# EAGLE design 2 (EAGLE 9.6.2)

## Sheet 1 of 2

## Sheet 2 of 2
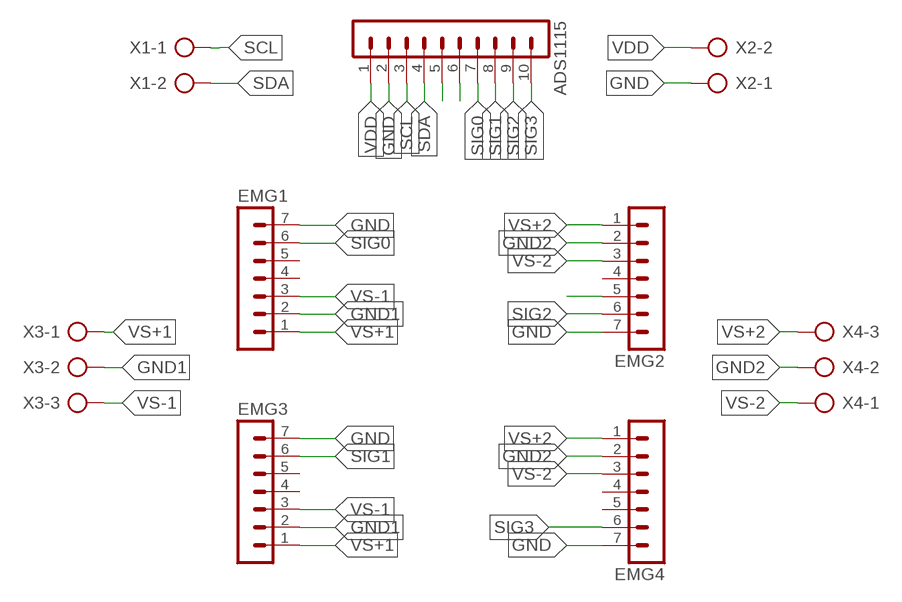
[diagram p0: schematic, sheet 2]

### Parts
ADS1115  MA10-1  [MA10-1]
EMG1  MA07-1  [MA07-1]
EMG2  MA07-1  [MA07-1]
EMG3  MA07-1  [MA07-1]
EMG4  MA07-1  [MA07-1]
X1  AK300/2  [AK300/2]
X2  AK300/2  [AK300/2]
X3  AK300/3  [AK300/3]
X4  AK300/3  [AK300/3]

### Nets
GND: ADS1115.2 EMG1.7 EMG2.7 EMG3.7 EMG4.7 X2.1
GND1: EMG1.2 EMG3.2 X3.2
GND2: EMG2.2 EMG4.2 X4.2
N$7: ADS1115.5
N$8: ADS1115.6
N$14: EMG2.5
SCL: ADS1115.3 X1.1
SDA: ADS1115.4 X1.2
SIG0: ADS1115.7 EMG1.6
SIG1: ADS1115.8 EMG3.6
SIG2: ADS1115.9 EMG2.6
SIG3: ADS1115.10 EMG4.6
VDD: ADS1115.1 X2.2
VS+1: EMG1.1 EMG3.1 X3.1
VS+2: EMG2.1 EMG4.1 X4.3
VS-1: EMG1.3 EMG3.3 X3.3
VS-2: EMG2.3 EMG4.3 X4.1
Unconnected: EMG1.4 EMG1.5 EMG2.4 EMG3.4 EMG3.5 EMG4.4 EMG4.5

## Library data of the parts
ADS1115 = con-lstb:MA10-1: PIN HEADER; OC_FARNELL: unknown; OC_NEWARK: unknown
EMG1-EMG4 = con-lstb:MA07-1: PIN HEADER; OC_FARNELL: unknown; OC_NEWARK: unknown
X1 X2 = con-ptr500:AK300/2: CONNECTOR; OC_FARNELL: unknown; OC_NEWARK: unknown
X3 X4 = con-ptr500:AK300/3: CONNECTOR; OC_FARNELL: unknown; OC_NEWARK: unknown

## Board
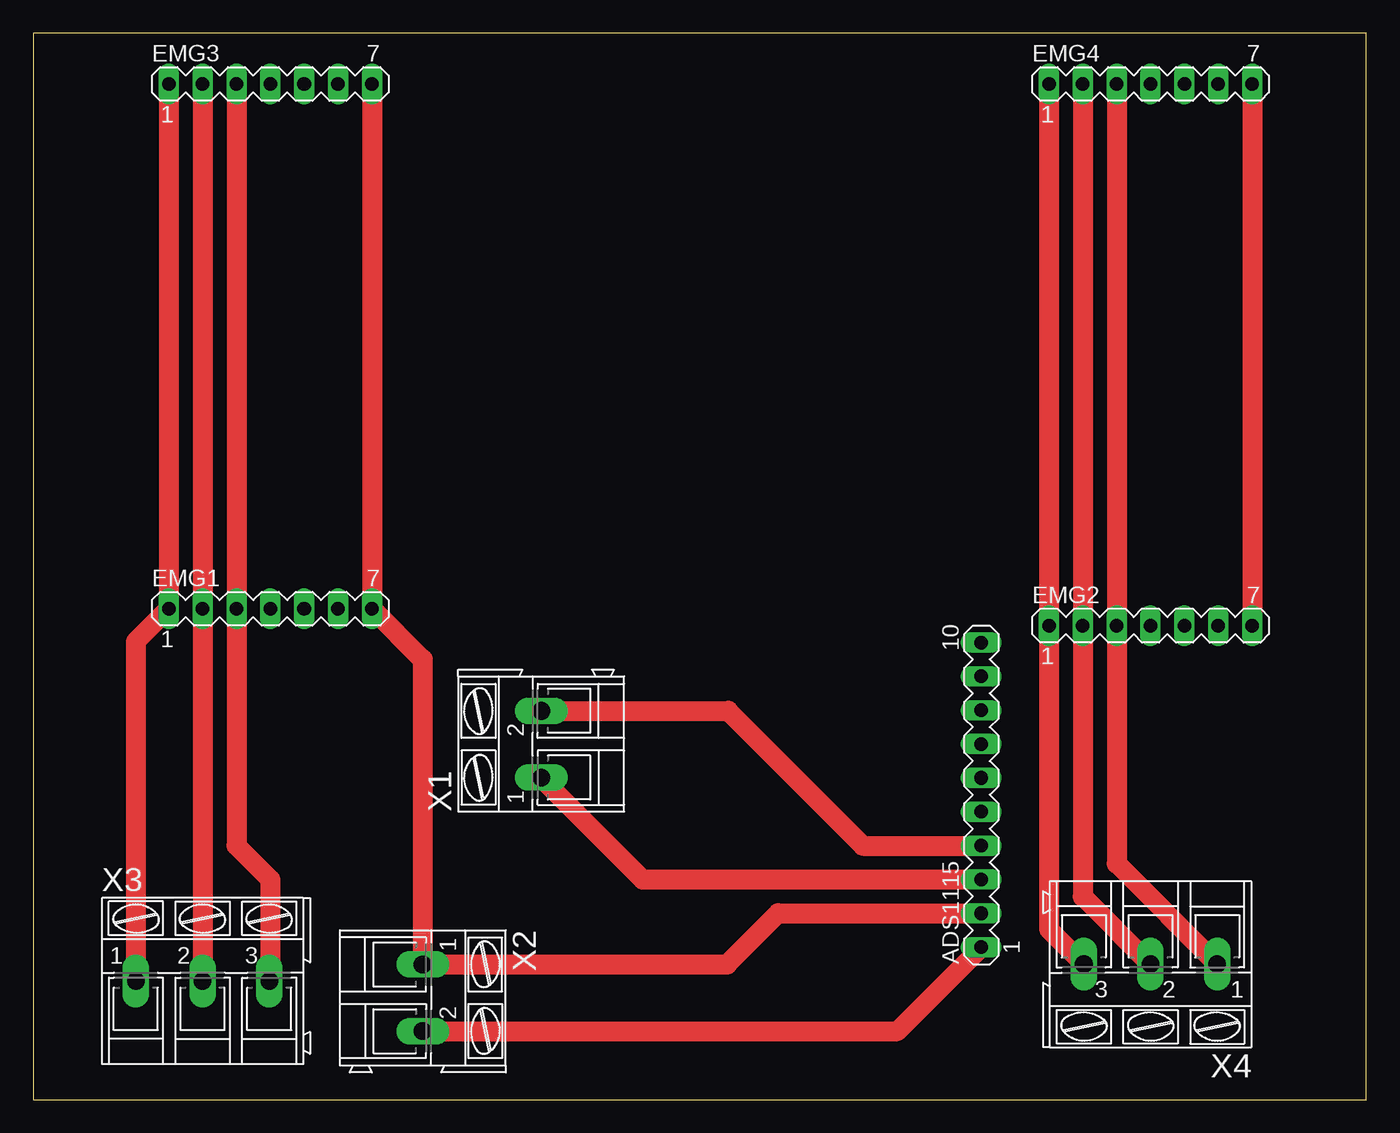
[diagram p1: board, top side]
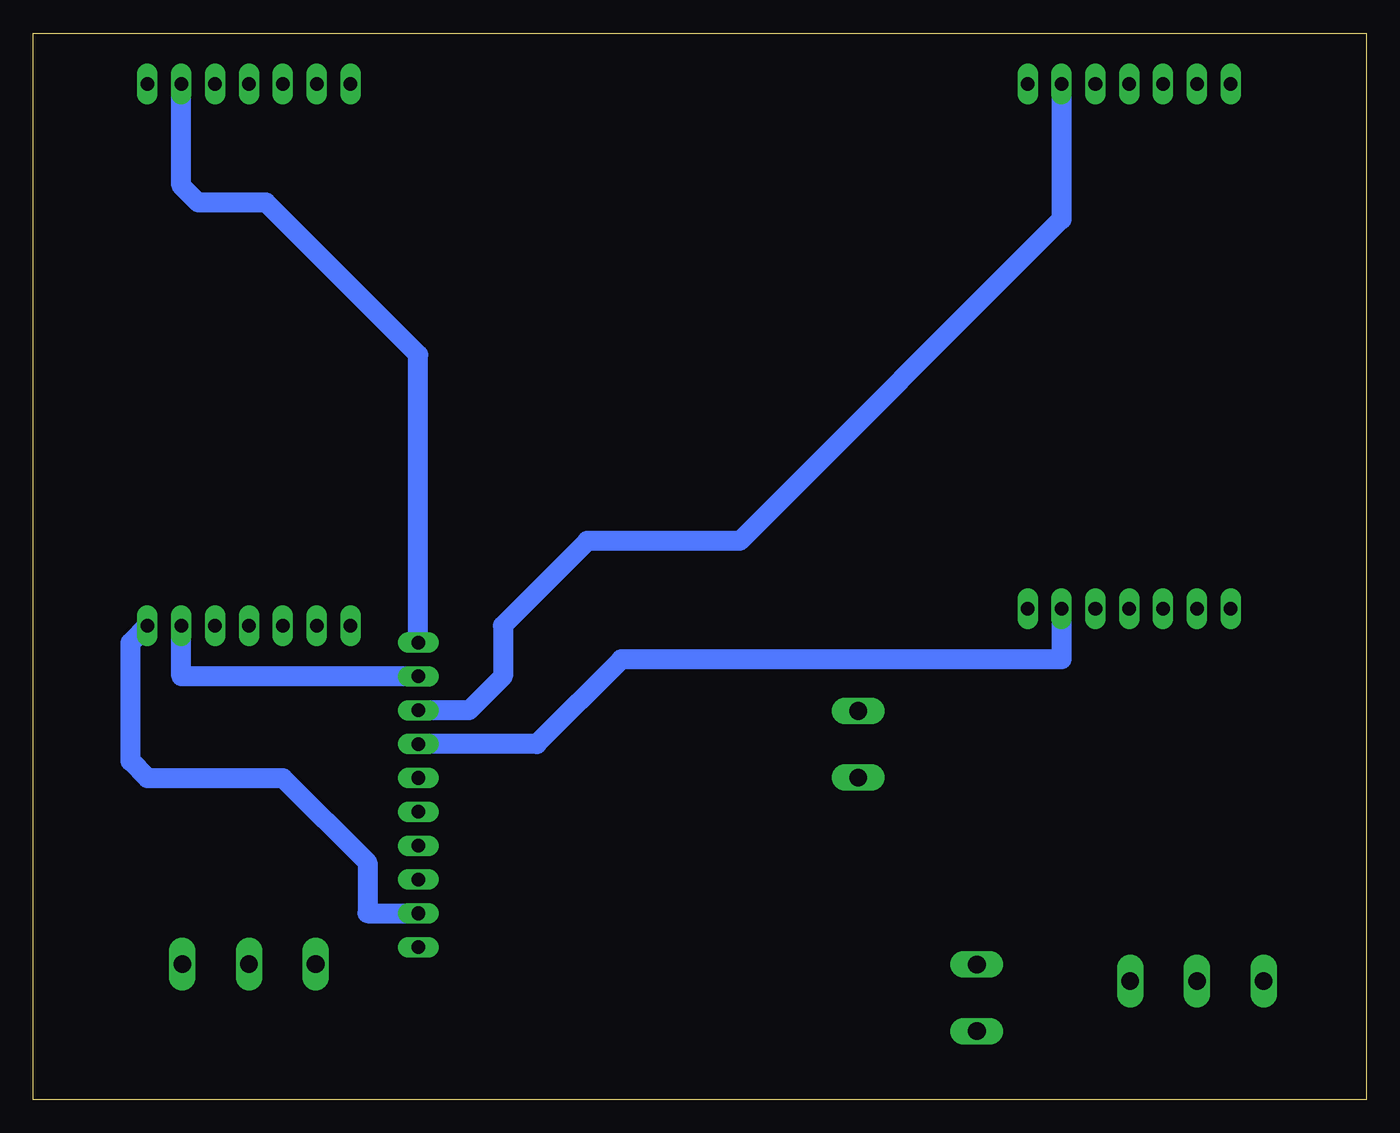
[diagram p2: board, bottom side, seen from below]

Size 100 x 80 mm. Coordinates in mm from the lower left corner, seen from the top.
Outline: 0,0 100,0 100,80 0,80 0,0
Copper layers (1*16): Top 0.035mm / dielectric 1.5mm / Bottom 0.035mm
Design rules "default": minimum track width 6mil, minimum drill 0.35mm, track to track 6mil, track to pad 6mil, pad to pad 6mil, via to via 6mil, smd to smd 6mil, copper to edge 40mil, drill to drill 6mil, minimum pad ring 10mil, minimum via ring 8mil, stop-mask expansion 4mil, vias tented up to drill 0mil, thermal gap 10mil

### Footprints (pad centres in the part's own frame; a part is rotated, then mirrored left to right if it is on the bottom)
MA10-1 = drill 1.016 long: 1 -11.43,0; 2 -8.89,0; 3 -6.35,0; 4 -3.81,0; 5 -1.27,0; 6 1.27,0; 7 3.81,0; 8 6.35,0; 9 8.89,0; 10 11.43,0
MA07-1 = drill 1.016 long: 1 -7.62,0; 2 -5.08,0; 3 -2.54,0; 4 0,0; 5 2.54,0; 6 5.08,0; 7 7.62,0
AK300/2 = drill 1.321 long: 1 -2.515,0; 2 2.489,0
AK300/3 = drill 1.321 long: 1 -5.004,0; 2 0,0; 3 5.004,0

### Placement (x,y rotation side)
ADS1115  71.12,22.86 90 top
EMG1  17.78,36.83 0 top
EMG2  83.82,35.56 0 top
EMG3  17.78,76.2 0 top
EMG4  83.82,76.2 0 top
X1  38.1,26.67 90 top
X2  29.21,7.62 270 top
X3  12.7,8.89 0 top
X4  83.82,10.16 180 top

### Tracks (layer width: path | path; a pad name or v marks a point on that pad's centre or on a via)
GND
  Top 1.5: EMG3.7 EMG1.7 29.21,33.02 X2.1 52.05,10.13 55.88,13.97 ADS1115.2 | EMG4.7 EMG2.7
  Bottom 1.5: EMG2.7 92.71,34.29 92.71,25.4 91.44,24.13 81.28,24.13 74.93,17.78 74.93,13.97 ADS1115.2
GND1
  Top 1.5: EMG3.2 EMG1.2 X3.2
GND2
  Top 1.5: X4.2 78.74,15.24 EMG2.2 EMG4.2
SCL
  Top 0.254: X1.1 38.1,24.13
  Top 1.5: 38.1,24.13 45.72,16.51 ADS1115.3
SDA
  Top 1.5: X1.2 52.12,29.16 62.23,19.05 ADS1115.4
SIG0
  Bottom 1.5: EMG1.6 22.86,33.02 55.88,33.02 62.23,26.67 ADS1115.7
SIG1
  Bottom 1.5: EMG3.6 22.86,66.04 46.99,41.91 58.42,41.91 64.77,35.56 64.77,31.75 67.31,29.21 ADS1115.8
SIG2
  Bottom 1.5: ADS1115.9 88.9,31.75 EMG2.6
SIG3
  Bottom 1.5: ADS1115.10 71.12,55.88 82.55,67.31 87.63,67.31 88.9,68.58 EMG4.6
VDD
  Top 1.5: X2.2 64.82,5.13 ADS1115.1
VS+1
  Top 1.5: EMG3.1 EMG1.1 7.7,34.37 X3.1
VS+2
  Top 1.5: X4.3 76.2,12.78 EMG2.1 EMG4.1
VS-1
  Top 0.254: 17.78,8.97 X3.3
  Top 1.5: EMG3.3 EMG1.3 15.24,19.05 17.78,16.51 17.78,8.97
VS-2
  Top 1.5: X4.1 81.28,17.7 EMG2.3 EMG4.3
